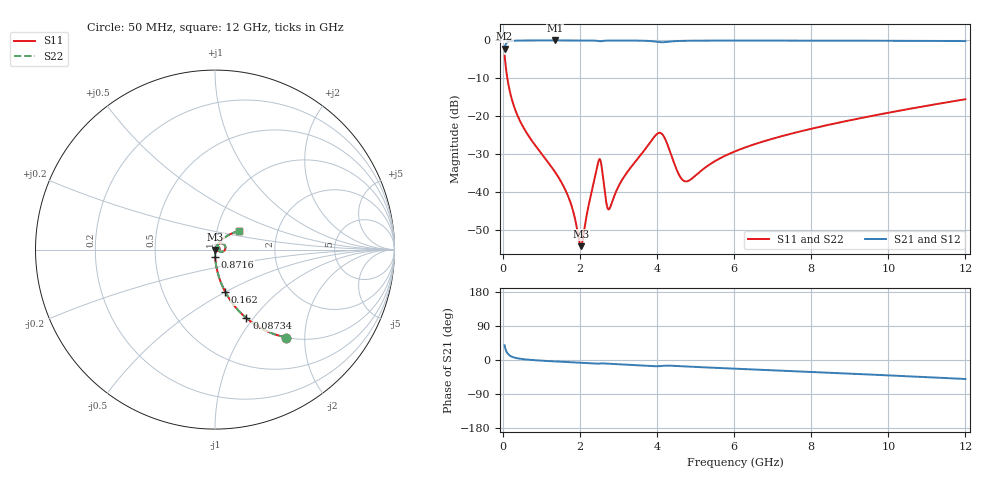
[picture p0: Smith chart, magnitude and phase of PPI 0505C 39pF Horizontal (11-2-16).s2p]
# MHz S MA R 50
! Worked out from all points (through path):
!   1601 points, 50 MHz to 12 GHz, reference 50 ohm
!   highest |S21| = -0.01 dB at 1.357 GHz (marker M1); lowest = -2.2 dB at 50 MHz (marker M2)
!   group delay of S21, straight-line fit = 12.4 ps
!   lowest |S11| = -54.4 dB at 2.029 GHz (marker M3), VSWR 1.00, Z = 50.2 - j0.0341 ohm
!   |S11| at or under -10 dB: 121.3 MHz to end of sweep
!   |S22| runs from -54.4 to -4.0 dB; largest |S21 - S12| = 0
!   S11 on the Smith chart (normalised r, x): 50 MHz: 1.00, -1.62; 87.34 MHz: 1.00, -0.92; 162 MHz: 1.00, -0.50; 871.6 MHz: 1.00, -0.08; 12 GHz: 1.27, +0.27
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50  0.6295 -51.1  0.7767 38.8  0.7767 38.8  0.6295 -51.1
87.34375  0.4204 -65.4  0.9069 24.6  0.9069 24.6  0.4204 -65.4
162.0312  0.2414 -76.5  0.9699 13.4  0.9699 13.4  0.2414 -76.5
415.9688  0.09362 -85.6  0.9948 3.9  0.9948 3.9  0.09362 -85.6
871.5625  0.03927 -89.3  0.9981 -0.8  0.9981 -0.8  0.03927 -89.3
1357.031  0.01825 -89.7  0.9984 -3.7  0.9984 -3.7  0.01825 -89.7
1730.469  0.007896 -84.5  0.9983 -5.7  0.9983 -5.7  0.007896 -84.5
2029.219  0.001911 -10.2  0.998 -7.2  0.998 -7.2  0.001911 -10.2
2044.156  0.001965 1.6  0.9979 -7.2  0.9979 -7.2  0.001965 1.6
2492.281  0.02598 26.4  0.9787 -9.7  0.9787 -9.7  0.02598 26.4
2559.5  0.02266 -11.8  0.9772 -9.0  0.9772 -9.0  0.02266 -11.8
2701.406  0.006602 -7.0  0.9932 -9.5  0.9932 -9.5  0.006602 -7.0
2768.625  0.005954 24.9  0.9949 -9.9  0.9949 -9.9  0.005954 24.9
3157  0.01605 64.5  0.9959 -12.0  0.9959 -12.0  0.01605 64.5
4038.312  0.05962 23.4  0.9532 -16.4  0.9532 -16.4  0.05962 23.4
4187.688  0.05287 -5.2  0.9476 -15.2  0.9476 -15.2  0.05287 -5.2
4553.656  0.01754 -13.1  0.9822 -16.0  0.9822 -16.0  0.01754 -13.1
4732.906  0.01373 13.1  0.9878 -17.0  0.9878 -17.0  0.01373 13.1
6025  0.03417 59.0  0.9942 -22.9  0.9942 -22.9  0.03417 59.0
8019.156  0.06828 54.8  0.9929 -31.6  0.9929 -31.6  0.06828 54.8
10013.31  0.111 47.0  0.9886 -40.6  0.9886 -40.6  0.111 47.0
12000  0.1669 38.1  0.98 -50.2  0.98 -50.2  0.1669 38.1
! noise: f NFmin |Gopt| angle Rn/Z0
50  0.0004336  0.8778  0.5729  0.000767
1372  0.004271  0.6927  4.913  0.002703
2701  0.01334  0.7952  9.514  0.01337
4031  0.04294  0.9001  14.14  0.09258
5360  0.01811  0.7173  18.66  0.01234
6682  0.01719  0.6473  22.98  0.008895
8012  0.01857  0.6193  27.22  0.008615
9341  0.02046  0.6056  31.35  0.008933
1.067e+04  0.0226  0.5996  35.35  0.009496
1.2e+04  0.02494  0.5986  39.22  0.01023
